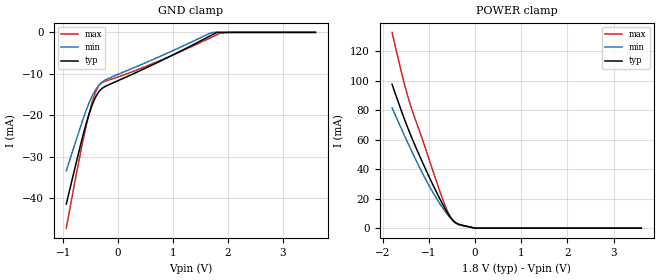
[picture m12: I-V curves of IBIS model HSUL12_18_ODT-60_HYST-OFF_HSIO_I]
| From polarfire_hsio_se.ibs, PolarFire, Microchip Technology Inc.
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|   HSUL12_18_ODT-60_HYST-OFF_HSIO_I
[Model]   HSUL12_18_ODT-60_HYST-OFF_HSIO_I
Model_type  Input
Vinl =   0.5
Vinh =   0.7
|   typ   min   max
C_comp_pullup   1.335e-12   1.335e-12   1.380e-12
C_comp_pulldown  1.335e-12   1.335e-12   1.380e-12
[Temperature Range]   25   100   -40
[Voltage Range]   1.8   1.71   1.89
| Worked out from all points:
|   POWER clamp passes 1 mA (typ) near -0.14 V on its own axis
[GND Clamp]
| Voltage   I(typ)   I(min)   I(max)
-945mV    -41.38mA   -33.35mA   -47.18mA
-767.8mV  -31.59mA   -26.09mA   -34.55mA
-649.7mV  -25.28mA   -21.3mA    -26.65mA
-531.6mV  -19.75mA   -17.07mA   -19.68mA
-413.4mV  -15.65mA   -13.87mA   -14.42mA
-354.4mV  -14.34mA   -12.77mA   -12.86mA
-295.3mV  -13.52mA   -11.99mA   -12.1mA
675mV     -7.529mA   -6.315mA   -7.286mA
1.688V    -784.6uA   -142uA     -1.28mA
1.8V      222.5nA    0A         -571.4uA
2.036V    0A         0A         0A
3.6V      0A         0A         0A
[POWER Clamp]
| Voltage   I(typ)   I(min)   I(max)
-1.8V     97.61mA    81.6mA     132.8mA
-1.536V   74.21mA    63.1mA     98.12mA
-1.417V   64.65mA    55.06mA    84.95mA
-1.358V   60.15mA    51.12mA    79.23mA
-1.004V   35.23mA    29.1mA     47.15mA
-767.8mV  19.97mA    16.63mA    25.11mA
-649.7mV  13.06mA    11.27mA    15.11mA
-531.6mV  7.219mA    6.708mA    7.173mA
-413.4mV  3.475mA    3.49mA     3.055mA
-295.3mV  2.087mA    1.956mA    1.887mA
0V        0A         86.3uA     0A
3.6V      0A         0A         0A
